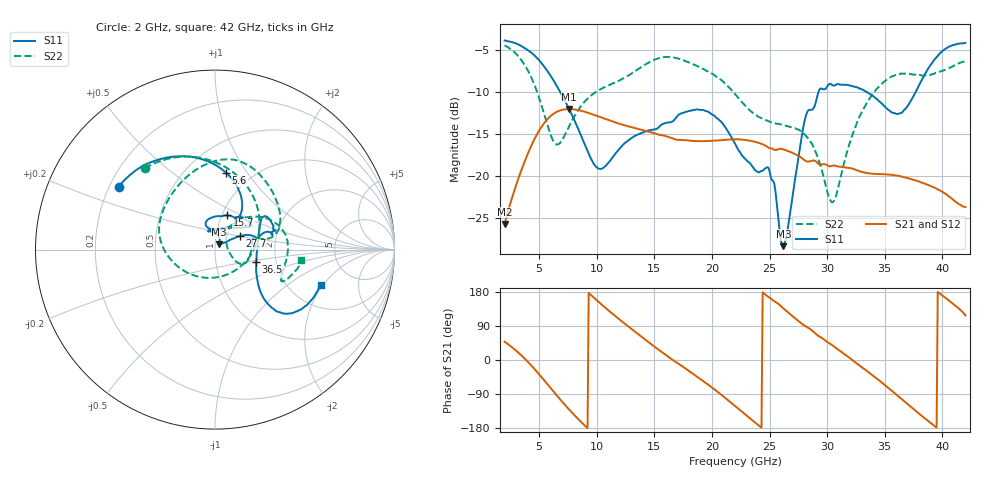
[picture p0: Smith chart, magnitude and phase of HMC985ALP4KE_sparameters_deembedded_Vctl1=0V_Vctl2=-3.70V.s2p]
!s2p File: Measurements: S11, S21, S12, S22
# GHz S dB R 50.0
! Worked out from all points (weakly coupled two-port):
!   401 points, 2 GHz to 42 GHz, reference 50 ohm
!   highest |S21| = -12.05 dB at 7.6 GHz (marker M1); lowest = -25.8 dB at 2 GHz (marker M2)
!   lowest |S11| = -28.4 dB at 26.2 GHz (marker M3), VSWR 1.08, Z = 52.3 + j3.13 ohm
!   |S11| at or under -10 dB: 6.819 GHz to 29.25 GHz (22.43 GHz wide, 124 % of centre); 33.42 GHz to 37.69 GHz (4.273 GHz wide, 12 % of centre)
!   |S22| runs from -23.2 to -4.4 dB; largest |S21 - S12| = 0.00022
!   S11 on the Smith chart (normalised r, x): 2 GHz: 0.24, +0.28; 5.6 GHz: 0.77, +0.81; 15.7 GHz: 1.06, +0.42; 27.7 GHz: 1.30, +0.20; 36.5 GHz: 1.57, -0.23; 42 GHz: 2.95, -1.89
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2  -3.86 146.9  -25.77 48.3  -25.77 48.3  -4.45 130.8
3.6  -4.64 120.1  -18.81 7.9  -18.82 7.9  -6.50 85.7
4.6  -5.66 101.3  -15.62 -23.9  -15.62 -23.9  -9.18 49.2
5.6  -7.28 81.7  -13.44 -59.6  -13.44 -59.6  -13.41 -1.6
6.5  -9.22 66.3  -12.40 -92.5  -12.40 -92.5  -16.27 -68.8
7.6  -12.05 54.5  -12.05 -130.6  -12.05 -130.7  -14.11 -137.8
8.7  -15.43 54.8  -12.27 -165.3  -12.28 -165.3  -11.57 -172.0
10.4  -19.19 90.1  -13.05 146.9  -13.05 146.9  -9.62 160.7
15.4  -14.19 75.6  -15.12 26.6  -15.12 26.5  -5.97 85.6
15.7  -13.86 70.3  -15.18 19.9  -15.19 19.9  -5.88 81.8
19.4  -12.25 33.2  -15.88 -58.9  -15.88 -58.9  -7.38 34.6
22  -16.17 51.4  -15.66 -121.2  -15.66 -121.2  -10.27 11.7
24.9  -19.06 104.5  -16.65 166.5  -16.64 166.5  -13.49 12.5
26.2  -28.42 52.0  -16.87 136.2  -16.87 136.2  -13.97 -3.9
27.7  -16.14 28.7  -17.80 98.0  -17.81 98.0  -14.67 -23.7
28.7  -12.12 12.6  -18.19 77.4  -18.19 77.4  -16.25 -29.8
30.5  -9.22 18.3  -18.81 37.8  -18.81 37.8  -23.18 17.7
32.8  -9.58 33.9  -19.46 -14.4  -19.46 -14.4  -12.98 49.6
35.4  -12.22 11.7  -19.88 -75.9  -19.88 -75.9  -8.34 19.4
36.5  -12.47 -16.7  -20.12 -103.9  -20.13 -104.0  -7.81 6.0
39.5  -5.86 -43.7  -21.56 -178.2  -21.56 -178.2  -7.72 -25.1
42  -4.15 -18.6  -23.74 117.4  -23.75 117.3  -6.29 -6.7
